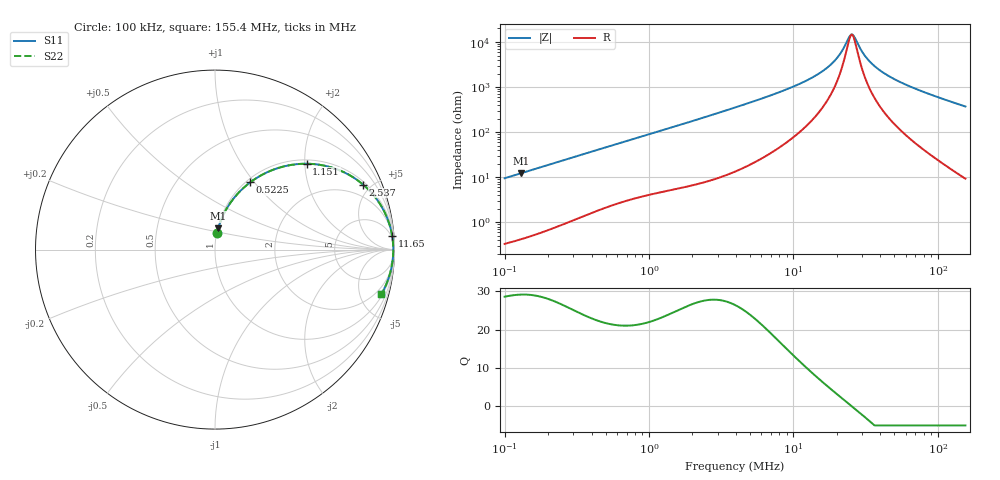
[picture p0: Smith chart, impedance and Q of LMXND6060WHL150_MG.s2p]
! LMXND6060WHL150_MG  S-PARAMETER MODEL  ( General Type )
! Model Generated by TAIYO YUDEN Corporation (https://www.yuden.co.jp/en/)
! Version 1.0
! TAIYO YUDEN Control No. 191025NI43SB-FBB
! Copyright(c) 2019 TAIYO YUDEN CO.,LTD. All Rights Reserved.
! Product Description (link to TY-COMPAS)
! https://ds.yuden.co.jp/TYCOMPAS/or/detail?pn=LMXND6060WHL150MMG&u=M
! Products Name : Inductors
! Characteristics :
!  Inductance : 15 uH , SRF(min) : 17 MHz , DC Resistance(max) : 0.1235 Ohm
!  Rated Current : Saturation :1600 mA , Temp Rise : 1800 mA (40 degC)
!  Case Size : 6.0 x 6.0 / 0.236 x 0.236 [mm/inch] , Thickness : 2.8 / 0.11 [mm/inch]
!  (Conditions: Temperature = 25 degC , DC Bias Current/Voltage = 0A / 0V)
! External Node Assignments :
!  1  o---GGG---o  2
! GND o---------o GND
! Frequency Range : 0.1MHz  -  155.401204MHz  [ 402 STEP ]
# MHz S RI R 50
! Freq[MHz].  S11 Real  S11 Imag  S21 Real  S21 Imag  S12 Real  S12 Imag  S22 Real  S22 Imag
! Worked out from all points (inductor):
!   401 points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, 100 kHz to 155.4 MHz, reference 50 ohm
!   read as one part in series: L = 15 uH near 103.7 kHz
!   highest Q = 29.2 at 129.3 kHz (marker M1), where L = 15 uH
!   self-resonance near 25.21 MHz
!   S11 on the Smith chart (normalised r, x): 100 kHz: 1.01, +0.19; 522.5 kHz: 1.04, +0.95; 1.151 MHz: 1.09, +2.04; 2.537 MHz: 1.16, +4.47; 11.65 MHz: 3, +25; 155.4 MHz: 1.18, -7.41
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0.1  0.0121 0.0931  0.9879 -0.0931  0.9879 -0.0931  0.0121 0.0931
0.12933  0.0186 0.1191  0.9814 -0.1191  0.9814 -0.1191  0.0186 0.1191
0.342427  0.101 0.2813  0.899 -0.2813  0.899 -0.2813  0.101 0.2813
0.522489  0.1967 0.375  0.8033 -0.375  0.8033 -0.375  0.1967 0.375
1.151221  0.511 0.4784  0.489 -0.4784  0.489 -0.4784  0.511 0.4784
1.172566  0.5196 0.4783  0.4804 -0.4783  0.4804 -0.4783  0.5196 0.4783
2.53653  0.8248 0.3625  0.1752 -0.3625  0.1752 -0.3625  0.8248 0.3625
3.942096  0.9169 0.2578  0.0831 -0.2578  0.0831 -0.2578  0.9169 0.2578
7.362085  0.9726 0.138  0.0274 -0.138  0.0274 -0.138  0.9726 0.138
11.65378  0.987 0.0764  0.013 -0.0764  0.013 -0.0764  0.987 0.0764
13.49882  0.9894 0.0601  0.0106 -0.0601  0.0106 -0.0601  0.9894 0.0601
16.52193  0.9916 0.0395  0.00843 -0.0395  0.00843 -0.0395  0.9916 0.0395
19.13771  0.9925 0.0256  0.00746 -0.0256  0.00746 -0.0256  0.9925 0.0256
20.97892  0.9929 0.0172  0.00706 -0.0172  0.00706 -0.0172  0.9929 0.0172
24.30033  0.9933 0.00393  0.00675 -0.00393  0.00675 -0.00393  0.9933 0.00393
25.2098  0.9933 0.000646  0.00672 -0.000646  0.00672 -0.000646  0.9933 0.000646
26.63823  0.9933 -0.00428  0.00673 0.00428  0.00673 0.00428  0.9933 -0.00428
30.29394  0.9931 -0.0159  0.00694 0.0159  0.00694 0.0159  0.9931 -0.0159
33.8242  0.9926 -0.026  0.00736 0.026  0.00736 0.026  0.9926 -0.026
46.22367  0.9901 -0.0566  0.0099 0.0566  0.0099 0.0566  0.9901 -0.0566
75.90801  0.9794 -0.117  0.0206 0.117  0.0206 0.117  0.9794 -0.117
155.4012  0.9267 -0.2484  0.0733 0.2484  0.0733 0.2484  0.9267 -0.2484
